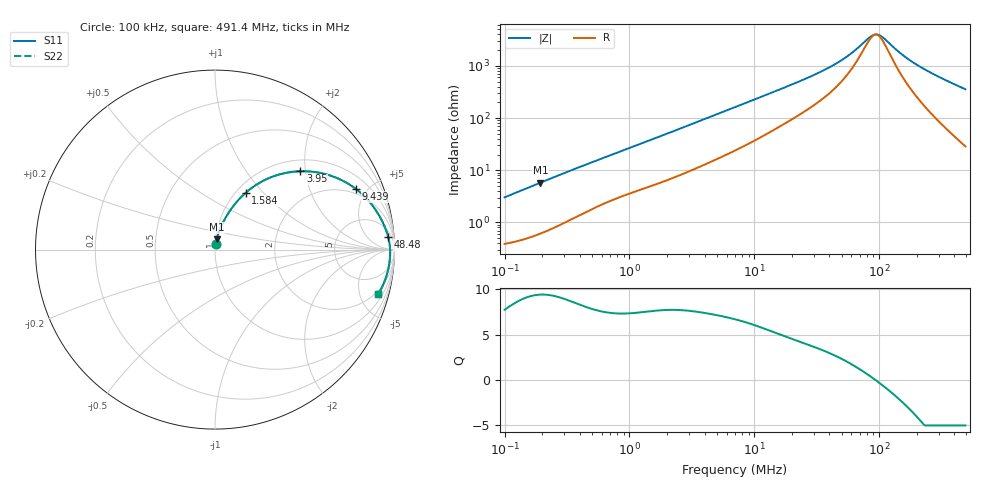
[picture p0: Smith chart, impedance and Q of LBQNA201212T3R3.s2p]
! LBQNA201212T3R3  S-PARAMETER MODEL  ( General Type )
! Model Generated by TAIYO YUDEN Corporation (http://www.ty-top.com)
! Version 1.0
! TAIYO YUDEN Control No. 191025NI43SB-FBB
! Copyright(c) 2019 TAIYO YUDEN CO.,LTD. All Rights Reserved.
! Product Description (link to TY-COMPAS)
! https://ds.yuden.co.jp/TYCOMPAS/or/detail?pn=LBQNA201212T3R3M&u=M
! Products Name : Inductors
! Characteristics :
!  Inductance : 3.3 uH , SRF(min) : 55 MHz , DC Resistance(max) : 0.39 Ohm
!  Rated Current : Saturation :330 mA , Temp Rise : 550 mA (20 degC)
!  Case Size : 2.0 x 1.25 / 0.079 x 0.049 [mm/inch] , Thickness : 1.25 / 0.049 [mm/inch]
!  (Conditions: Temperature = 25 degC , DC Bias Current/Voltage = 0A / 0V)
! External Node Assignments :
!  1  o---GGG---o  2
! GND o---------o GND
! Frequency Range : 0.1MHz  -  491.415554MHz  [ 402 STEP ]
# MHz S RI R 50
! Freq[MHz].  S11 Real  S11 Imag  S21 Real  S21 Imag  S12 Real  S12 Imag  S22 Real  S22 Imag
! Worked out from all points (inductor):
!   401 points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, 100 kHz to 491.4 MHz, reference 50 ohm
!   read as one part in series: L = 4.77 uH near 104.3 kHz
!   highest Q = 9.43 at 193.2 kHz (marker M1), where L = 4.73 uH
!   self-resonance near 93.8 MHz
!   S11 on the Smith chart (normalised r, x): 100 kHz: 1.01, +0.06; 1.584 MHz: 1.10, +0.80; 3.95 MHz: 1.25, +1.88; 9.439 MHz: 1.68, +4.23; 48.48 MHz: 10, +23; 491.4 MHz: 1.57, -7.11
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0.1  0.00475 0.0298  0.9952 -0.0298  0.9952 -0.0298  0.00475 0.0298
0.193236  0.00929 0.0566  0.9907 -0.0566  0.9907 -0.0566  0.00929 0.0566
0.415258  0.0276 0.1139  0.9724 -0.1139  0.9724 -0.1139  0.0276 0.1139
0.892376  0.08 0.2115  0.92 -0.2115  0.92 -0.2115  0.08 0.2115
1.583875  0.1701 0.3159  0.8299 -0.3159  0.8299 -0.3159  0.1701 0.3159
1.72439  0.1898 0.3324  0.8102 -0.3324  0.8102 -0.3324  0.1898 0.3324
2.752105  0.3333 0.4108  0.6667 -0.4108  0.6667 -0.4108  0.3333 0.4108
3.949587  0.4756 0.4365  0.5244 -0.4365  0.5244 -0.4365  0.4756 0.4365
7.010104  0.6974 0.3909  0.3026 -0.3909  0.3026 -0.3909  0.6974 0.3909
9.438982  0.7859 0.3373  0.2141 -0.3373  0.2141 -0.3373  0.7859 0.3373
15.71854  0.8843 0.2363  0.1157 -0.2363  0.1157 -0.2363  0.8843 0.2363
29.11  0.9422 0.1353  0.0578 -0.1353  0.0578 -0.1353  0.9422 0.1353
48.47626  0.9648 0.0707  0.0352 -0.0707  0.0352 -0.0707  0.9648 0.0707
59.9536  0.9701 0.047  0.0299 -0.047  0.0299 -0.047  0.9701 0.047
82.46025  0.9747 0.0134  0.0253 -0.0134  0.0253 -0.0134  0.9747 0.0134
89.77577  0.9754 0.00456  0.0246 -0.00456  0.0246 -0.00456  0.9754 0.00456
101.9837  0.9759 -0.00874  0.0241 0.00874  0.0241 0.00874  0.9759 -0.00874
120.8815  0.9759 -0.0269  0.0241 0.0269  0.0241 0.0269  0.9759 -0.0269
155.9923  0.9741 -0.0557  0.0259 0.0557  0.0259 0.0557  0.9741 -0.0557
210.041  0.9686 -0.0938  0.0314 0.0938  0.0314 0.0938  0.9686 -0.0938
314.5197  0.9519 -0.1573  0.0481 0.1573  0.0481 0.1573  0.9519 -0.1573
491.4156  0.91 -0.2487  0.09 0.2487  0.09 0.2487  0.91 -0.2487
